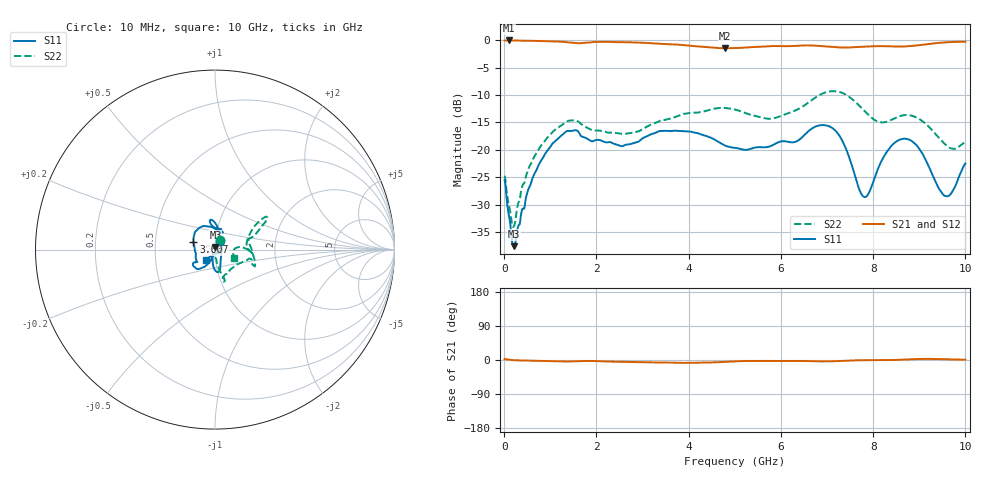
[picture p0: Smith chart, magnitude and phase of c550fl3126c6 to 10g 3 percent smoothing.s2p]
!Agilent Technologies,N5234A,MY52241123,A.10.00.00
!Agilent N5234A: A.10.00.00
!Date: Tuesday, April 23, 2019 10:30:54
!Correction: S11(Full 2 Port(1,2))
!S21(Full 2 Port(1,2))
!S12(Full 2 Port(1,2))
!S22(Full 2 Port(1,2))
!S2P File: Measurements: S11, S21, S12, S22:
# Hz S  dB  R 50
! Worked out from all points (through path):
!   1001 points, 10 MHz to 10 GHz, reference 50 ohm
!   highest |S21| = -0.07 dB at 99.91 MHz (marker M1); lowest = -1.5 dB at 4.785 GHz (marker M2)
!   lowest |S11| = -37.5 dB at 209.8 MHz (marker M3), VSWR 1.03, Z = 50.2 + j1.32 ohm
!   |S11| at or under -10 dB: start of sweep to end of sweep
!   |S22| runs from -34.0 to -9.3 dB; largest |S21 - S12| = 0.0012
!   S11 on the Smith chart (normalised r, x): 10 MHz: 1.05, +0.10; 3.007 GHz: 0.78, +0.07; 10 GHz: 0.90, -0.10
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1e7  -25.51 61.7  -0.07 2.5  -0.06 2.5  -24.69 62.7
9.991e7  -31.81 -75.0  -0.07 0.9  -0.06 0.9  -30.03 5.4
2.098e8  -37.54 80.7  -0.08 -0.6  -0.08 -0.6  -33.96 -62.2
5.1949e8  -27.32 -109.5  -0.12 -1.6  -0.12 -1.6  -23.60 -82.3
8.8912e8  -20.71 -117.1  -0.19 -2.6  -0.19 -2.6  -18.29 -76.8
1.34866e9  -16.63 -132.7  -0.37 -4.0  -0.37 -4.0  -14.88 -72.4
1.67833e9  -17.55 -147.5  -0.54 -2.7  -0.54 -2.7  -15.37 -76.0
2.53747e9  -19.32 -168.1  -0.39 -4.7  -0.38 -4.7  -17.06 -52.6
3.007e9  -17.86 160.8  -0.48 -6.2  -0.47 -6.2  -16.18 -30.1
3.34666e9  -16.63 139.6  -0.67 -6.9  -0.67 -6.9  -14.81 -19.8
4.04596e9  -16.68 116.5  -1.05 -7.5  -1.04 -7.5  -13.24 -17.8
4.78522e9  -19.19 85.0  -1.49 -4.8  -1.48 -4.8  -12.36 -22.1
5.005e9  -19.63 75.6  -1.45 -3.6  -1.45 -3.6  -12.66 -17.2
5.8042e9  -19.21 70.2  -1.09 -2.4  -1.09 -2.4  -14.31 14.6
6.67333e9  -16.11 100.4  -0.98 -3.3  -0.98 -3.3  -10.90 25.7
7.23277e9  -16.99 87.6  -1.32 -2.9  -1.32 -2.9  -9.38 32.7
7.81219e9  -28.59 4.6  -1.19 -0.5  -1.19 -0.5  -12.90 26.9
8.34166e9  -19.85 -72.9  -1.14 -0.4  -1.13 -0.4  -14.73 1.2
8.61139e9  -18.05 -80.1  -1.17 0.8  -1.17 0.7  -13.77 -4.7
8.87113e9  -18.61 -88.8  -1.04 2.2  -1.04 2.2  -13.87 -4.0
9.58042e9  -28.42 -114.7  -0.41 1.9  -0.40 1.9  -19.12 2.7
1e10  -22.47 -131.3  -0.29 0.7  -0.29 0.7  -18.52 -24.5
